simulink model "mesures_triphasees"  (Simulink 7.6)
settings: Solver=ode23tb  StartTime=0.0  StopTime=0.02  RelTol=1e-3
InitFcn:
  | clc
StopFcn:
  | close all
  | load Mesures_phases.mat
  | plot(x(1,:),x(2,:))
  | hold on
  | plot(x(1,:),x(3,:))
  | plot(x(1,:),x(4,:))
  | %axis([0 0.04 -20 1020])
  | grid
  | title('Tensions aux bornes de la charge sur les voies A, B et C')
  | xlabel('temps')
libraries: powerlib x12, simulink x1

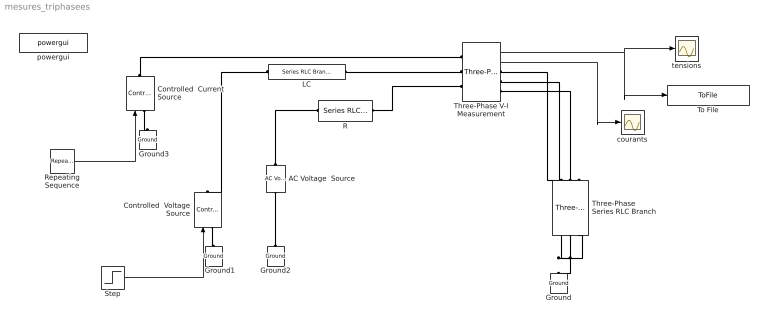
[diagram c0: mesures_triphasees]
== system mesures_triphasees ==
  AC Voltage  Source : powerlib/Electrical Sources/AC Voltage Source  DialogController=POWERSYS.PowerSysDialog  SystemSampleTime=-1  Amplitude=10  Phase=0  Frequency=60  SampleTime=0  Measurements=None
  Controlled  Current Source : powerlib/Electrical Sources/Controlled Current Source  DialogController=POWERSYS.PowerSysDialog  SystemSampleTime=-1  Initialize=on  Source_Type=AC  Amplitude=0  Phase=0  Frequency=0  Measurements=None
  Controlled  Voltage Source : powerlib/Electrical Sources/Controlled Voltage Source  DialogController=POWERSYS.PowerSysDialog  SystemSampleTime=-1  Initialize=on  Source_Type=AC  Amplitude=0  Phase=0  Frequency=0  Measurements=None
  Ground{,1..3} (4 alike) : powerlib/Elements/Ground  DialogController=POWERSYS.PowerSysDialog  PhysicalDomain=powersysdomain  SubClassName=unknown  LeftPortType=p1  RightPortType=p1  LConnTagsString=a
  LC : powerlib/Elements/Series RLC Branch  DialogController=POWERSYS.PowerSysDialog  PhysicalDomain=powersysdomain  SubClassName=unknown  LeftPortType=p1  RightPortType=p1  LConnTagsString=__new0  RConnTagsString=__new0  BranchType=LC  Resistance=10  Inductance=0.001  SetiL0=off  InitialCurrent=0  Capacitance=1e-3  Setx0=off  InitialVoltage=0  Measurements=None
  R : powerlib/Elements/Series RLC Branch  DialogController=POWERSYS.PowerSysDialog  PhysicalDomain=powersysdomain  SubClassName=unknown  LeftPortType=p1  RightPortType=p1  LConnTagsString=__new0  RConnTagsString=__new0  BranchType=R  Resistance=1  Inductance=1e-3  SetiL0=off  InitialCurrent=0  Capacitance=1e-6  Setx0=off  InitialVoltage=0  Measurements=None
  Repeating Sequence : simulink/Sources/Repeating Sequence  SystemSampleTime=-1  rep_seq_t=[0 0.005 0.01]  rep_seq_y=[0 4 0]
  Step : Step  Time=0.005  After=10  SampleTime=0
  Three-Phase Series RLC Branch : powerlib/Elements/Three-Phase Series RLC Branch  DialogController=POWERSYS.PowerSysDialog  PhysicalDomain=powersysdomain  SubClassName=unknown  LeftPortType=p1  RightPortType=p1  LConnTagsString=A|B|C  RConnTagsString=A|B|C  BranchType=R  Resistance=1  Inductance=1e-3  Capacitance=1e-6  Measurements=None
  Three-Phase V-I Measurement : powerlib/Measurements/Three-Phase V-I Measurement  DialogController=POWERSYS.PowerSysDialog  SystemSampleTime=-1  VoltageMeasurement=phase-to-ground  SetLabelV=off  LabelV=Vabc  Vpu=off  VpuLL=off  CurrentMeasurement=yes  SetLabelI=off  LabelI=Iabc  Ipu=off  Pbase=100e6  Vbase=500e3  OutputType=Complex  PhasorSimulation=off  PSBequivalent=0
  To File : ToFile  Filename=Mesures_phases.mat  MatrixName=x
  courants : Scope
  powergui : powerlib/powergui  Priority=2  SystemSampleTime=-1  SimulationMode=Continuous  SampleTime=0  frequency=60  SPID=off  DisableSnubberDevices=off  DisableRonSwitches=off  DisableVfSwitches=off  SwTol=0  Interpol=off  frequencyindice=60  echomessages=off  HookPort=off  DisplayEquations=off  FunctionMessages=off  EnableUseOfTLC=off  x0status=blocks  RestoreLinks=warning  ResistiveCurrentMeasurement=off  Frange=logspace(0,3,50)  Ylog=off  Xlog=off  ShowGrid=off  save=off  variable=ZData  ZoomFFT=on  StartTime=0.0  cycles=1  DisplayStyle=off  fundamental=60  FreqAxis=off  MaxFrequency=1000  frequencyindicesteady=1  RmsSteady=1  display=off  Ts=0  methode=off
  tensions : Scope
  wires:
  Three-Phase V-I Measurement/1 -> tensions/1, To File/1
  Step/1 -> Controlled  Voltage Source/1
  Repeating Sequence/1 -> Controlled  Current Source/1
  Three-Phase V-I Measurement/2 -> courants/1
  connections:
  R/RConn1 -- Three-Phase V-I Measurement/LConn3
  Three-Phase V-I Measurement/RConn3 -- Three-Phase Series RLC Branch/RConn3
  Three-Phase V-I Measurement/RConn2 -- Three-Phase Series RLC Branch/RConn2
  Three-Phase V-I Measurement/RConn1 -- Three-Phase Series RLC Branch/RConn1
  LC/RConn1 -- Three-Phase V-I Measurement/LConn2
  Three-Phase Series RLC Branch/LConn1 -- Ground/LConn1 -- Three-Phase Series RLC Branch/LConn2 -- Three-Phase Series RLC Branch/LConn3
  LC/LConn1 -- Controlled  Voltage Source/RConn1
  Controlled  Voltage Source/LConn1 -- Ground1/LConn1
  AC Voltage  Source/RConn1 -- R/LConn1
  AC Voltage  Source/LConn1 -- Ground2/LConn1
  Controlled  Current Source/LConn1 -- Ground3/LConn1
  Controlled  Current Source/RConn1 -- Three-Phase V-I Measurement/LConn1
